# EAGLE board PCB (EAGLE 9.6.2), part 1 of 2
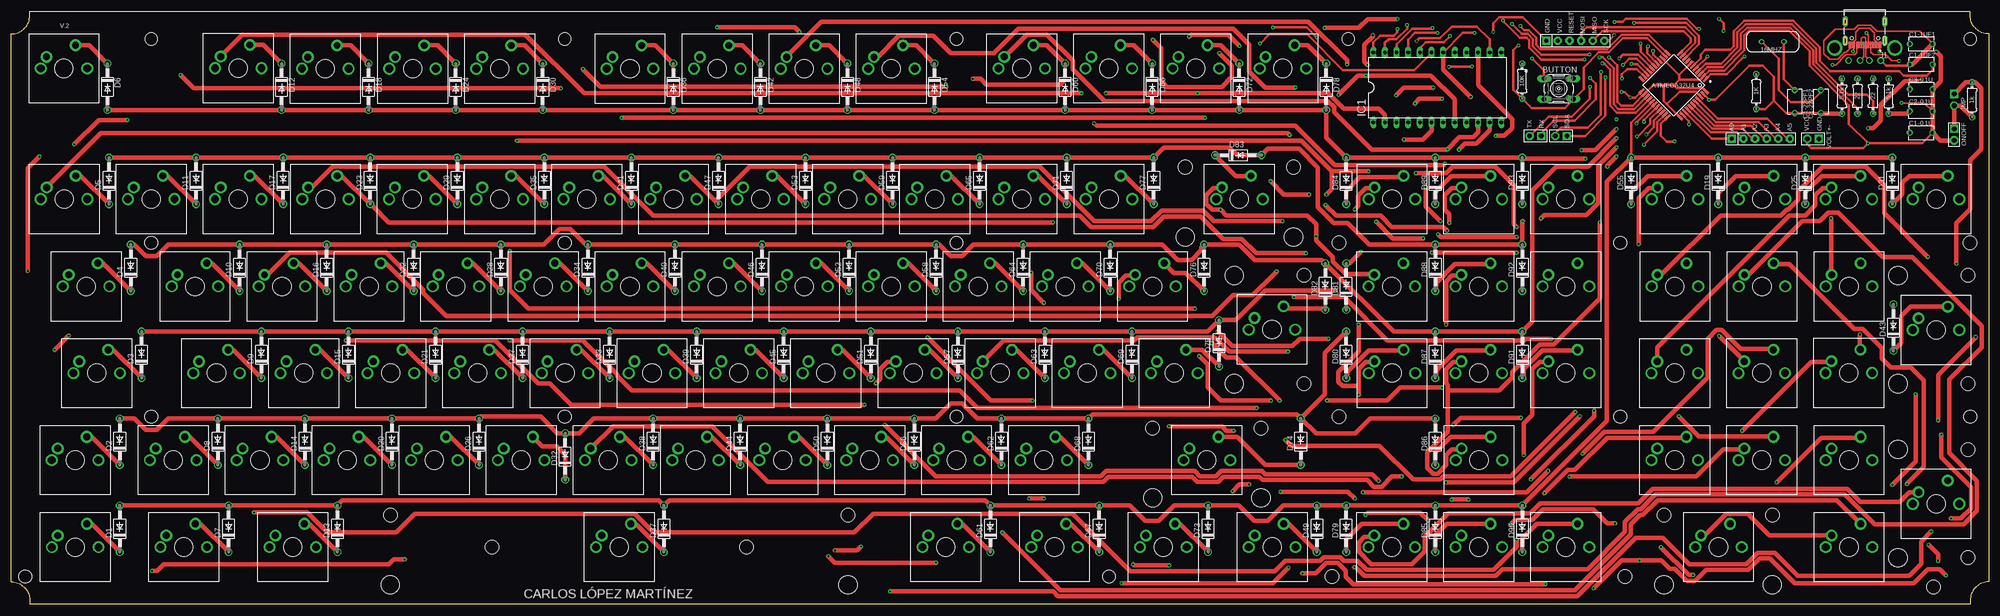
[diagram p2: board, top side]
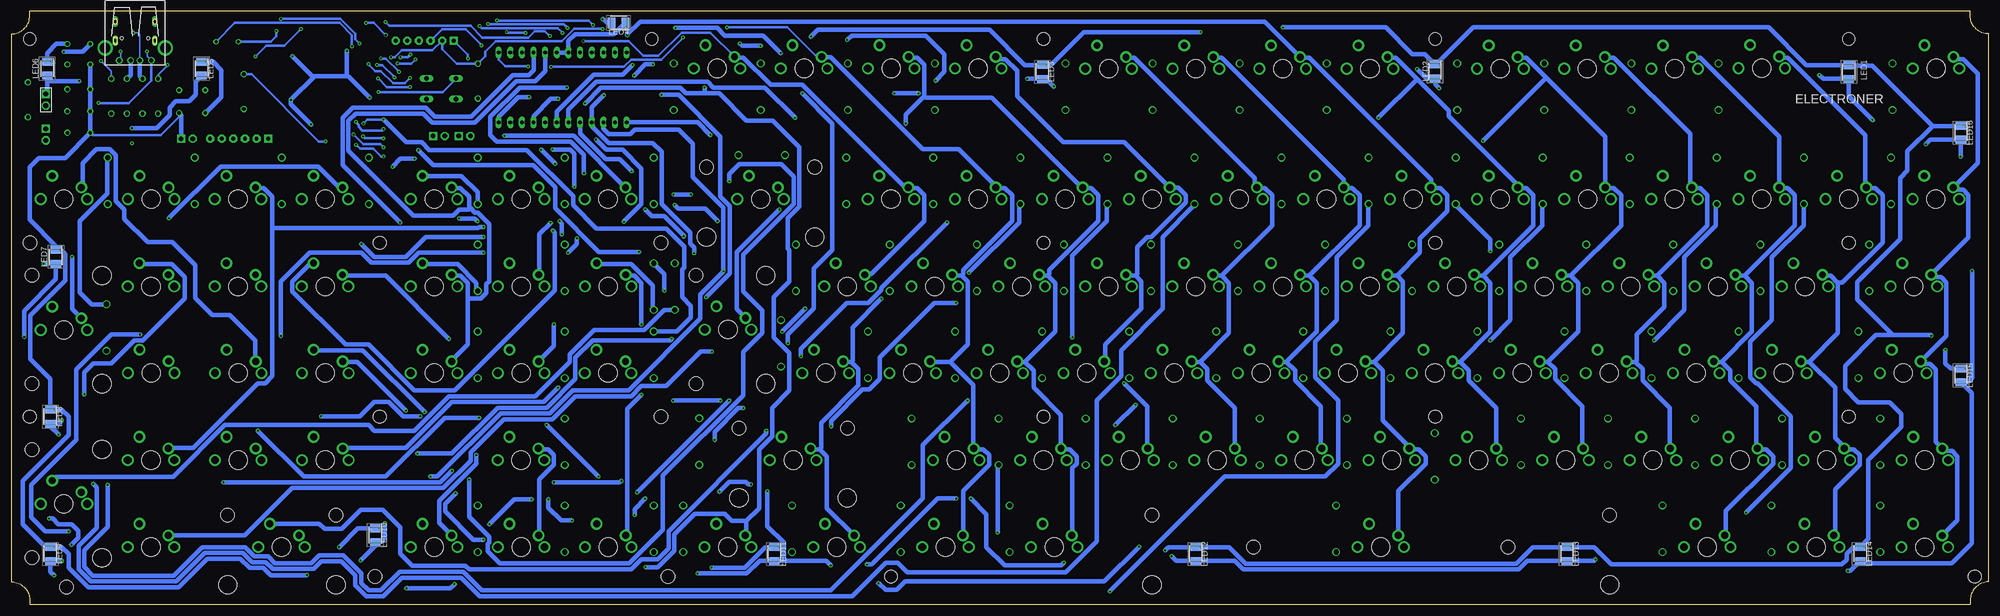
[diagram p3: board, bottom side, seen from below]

Size 431.5 x 129.5 mm. Coordinates in mm from the lower left corner, seen from the top.
Outline: 431.5,124.6 431.5,4.9 arc90 427.5,0.9 427.5,0 4,0 4,0.9 arc90 0,4.9 0,124.6 arc90 4,128.6 4,129.5 427.5,129.5 427.5,128.6 arc90 431.5,124.6
Copper layers (1*16): Top 0.035mm / dielectric 1.5mm / Bottom 0.035mm
Design rules "default *": minimum track width 0.3mm, minimum drill 0.35mm, track to track 3mil, track to pad 3mil, pad to pad 7mil, via to via 10mil, smd to smd 3mil, copper to edge 14mil, drill to drill 4mil, minimum pad ring 10mil, minimum via ring 8mil, stop-mask expansion 4mil, vias tented up to drill 0mil, thermal gap 10mil
Net classes: 0 default: width 0.203 mm
Holes 2.75 mm at 30.5,123.47 120.75,123.47 206.25,123.46 291.75,123.46 427.5,123.47
Holes 2.8 mm at 351.13,79 427.5,41 351.13,41 239.5,6.04 3,6.03 30.51,78.99 120.75,79 206.25,78.99 206.26,41 120.76,41 30.5,40.99
Holes 3 mm at 82.7,19.5 182.55,19.5 384.32,19.5 360.68,19.5 427,33.82 427,10.18 427,48.18 427,71.83 272.7,38.5 249.05,38.5 282.13,48.18 282.12,71.83 279.82,95.5 256.18,95.5 289.75,78.99 419.5,3.78 352.16,6.04 288.19,6.04 289.75,41 160.43,12.5 104.83,12.5 427.5,79
Holes 4 mm at 82.7,4.25 182.57,4.25 384.32,4.25 360.68,4.24 411.74,10.17 411.74,33.82 411.74,48.18 411.75,71.82 272.7,23.25 249.05,23.25 266.87,48.18 266.87,71.83 256.18,80.25 279.82,80.24

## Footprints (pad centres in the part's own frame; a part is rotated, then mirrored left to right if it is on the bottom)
SIP-100-06-32 = drill 0.813 pad 1.778 square: 1 -6.35,0 | drill 0.813 pad 1.778 octagon: 2 -3.81,0; 3 -1.27,0; 4 1.27,0; 5 3.81,0; 6 6.35,0
B3F-10XX = drill 1.016 long: 1 -3.251,2.261; 2 3.251,2.261; 3 -3.251,-2.261; 4 3.251,-2.261
CAP_RDE5C1H273J2M1H03A = drill 0.75 pad 1.15: 1 -2.5,0; 2 2.5,0
DO41-10 = drill 1.118: A 5.08,0; C -5.08,0
CHERRY-MX = drill 1.714 pad 1.93: P$3 -5.08,0; P$4 5.08,0 | drill 1.5 pad 2.54: SW1 -3.81,2.54; SW2 2.54,5.08 | hole 4: 0,0
DIL24-6 = drill 0.813 long: 1 -13.97,-7.62; 2 -11.43,-7.62; 3 -8.89,-7.62; 4 -6.35,-7.62; 5 -3.81,-7.62; 6 -1.27,-7.62; 7 1.27,-7.62; 8 3.81,-7.62; 9 6.35,-7.62; 10 8.89,-7.62; 11 11.43,-7.62; 12 13.97,-7.62; 13 13.97,7.62; 14 11.43,7.62; 15 8.89,7.62; 16 6.35,7.62; 17 3.81,7.62; 18 1.27,7.62; 19 -1.27,7.62; 20 -3.81,7.62; 21 -6.35,7.62; 22 -8.89,7.62; 23 -11.43,7.62; 24 -13.97,7.62
HRO_TYPE-C-31-M-12 = smd 0.6 x 1.45: A1B12 -3.25,5.095; A4B9 -2.45,5.095; B1A12 3.25,5.095; B4A9 2.45,5.095 | smd 0.3 x 1.45: A5 -1.25,5.095; A6 -0.25,5.095; A7 0.25,5.095; A8 1.25,5.095; B5 1.75,5.095; B6 0.75,5.095; B7 -0.75,5.095; B8 -1.75,5.095 | drill 0.65 pad 1.05 long: S1 -4.32,4.18; S2 4.32,4.18; S3 -4.32,0; S4 4.32,0 | hole 0.7: -2.89,3.65; 2.89,3.65
LEDM3528X200N = smd 1.65 x 2.25: 1 -1.5,0; 2 1.5,0
SIP-100-02-40 = drill 1.016 pad 1.778 square: 1 -1.27,0 | drill 1.016 pad 1.778 octagon: 2 1.27,0
0204/7 = drill 0.813 octagon: 1 -3.81,0; 2 3.81,0
QFP80P1200X1200X120-44N = smd 1.5 x 0.5: 1 -5.9,4; 2 -5.9,3.2; 3 -5.9,2.4; 4 -5.9,1.6; 5 -5.9,0.8; 6 -5.9,0; 7 -5.9,-0.8; 8 -5.9,-1.6; 9 -5.9,-2.4; 10 -5.9,-3.2; 11 -5.9,-4; 23 5.9,-4; 24 5.9,-3.2; 25 5.9,-2.4; 26 5.9,-1.6; 27 5.9,-0.8; 28 5.9,0; 29 5.9,0.8; 30 5.9,1.6; 31 5.9,2.4; 32 5.9,3.2; 33 5.9,4 | smd 0.5 x 1.5: 12 -4,-5.9; 13 -3.2,-5.9; 14 -2.4,-5.9; 15 -1.6,-5.9; 16 -0.8,-5.9; 17 0,-5.9; 18 0.8,-5.9; 19 1.6,-5.9; 20 2.4,-5.9; 21 3.2,-5.9; 22 4,-5.9; 34 4,5.9; 35 3.2,5.9; 36 2.4,5.9; 37 1.6,5.9; 38 0.8,5.9; 39 0,5.9; 40 -0.8,5.9; 41 -1.6,5.9; 42 -2.4,5.9; 43 -3.2,5.9; 44 -4,5.9
USB-A-H = drill 0.914: D+ 2.718,-1.003; D- 2.718,1.003; GND 2.718,-3.493; VBUS 2.718,3.493 | drill 2.311: P$5 0,-6.566; P$6 0,6.566
XTAL_ECS-160-20-4X = drill 0.63 pad 1.03: 1 -2.44,0; 2 2.44,0

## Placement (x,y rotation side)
ANALOG  Boot  [SIP-100-06-32]  381.8,101.7 0 top
BUTTON  [B3F-10XX]  337.7,112.6 0 top
C1-0.1U  RDE5C1H273J2M1H03A  [CAP_RDE5C1H273J2M1H03A]  416.8,103 180 top
C1-1UF1  RDE5C1H273J2M1H03A  [CAP_RDE5C1H273J2M1H03A]  416.8,122.4 0 top
C1-1UF2  RDE5C1H273J2M1H03A  [CAP_RDE5C1H273J2M1H03A]  416.8,117.9 180 top
C1-22PF1  RDE5C1H273J2M1H03A  [CAP_RDE5C1H273J2M1H03A]  389.2,109.8 270 top
C1-22PF2  RDE5C1H273J2M1H03A  [CAP_RDE5C1H273J2M1H03A]  394.9,109.8 270 top
C2-0.1U  RDE5C1H273J2M1H03A  [CAP_RDE5C1H273J2M1H03A]  416.8,107.7 180 top
C3-0.1U  RDE5C1H273J2M1H03A  [CAP_RDE5C1H273J2M1H03A]  416.8,112.5 180 top
D1  1N4004  [DO41-10]  23.65,16.5 90 top
D2  1N4004  [DO41-10]  23.65,35.5 90 top
D3  1N4004  [DO41-10]  28.4,54.5 90 top
D4  1N4004  [DO41-10]  26.05,73.5 90 top
D5  1N4004  [DO41-10]  21.3,92.5 90 top
D6  1N4004  [DO41-10]  20.95,113.05 270 top
D7  1N4004  [DO41-10]  47.4,16.5 90 top
D8  1N4004  [DO41-10]  45.05,35.5 90 top
D9  1N4004  [DO41-10]  54.55,54.5 90 top
D10  1N4004  [DO41-10]  49.8,73.5 90 top
D11  1N4004  [DO41-10]  40.3,92.5 90 top
D12  1N4004  [DO41-10]  58.95,113.05 270 top
D13  1N4004  [DO41-10]  71.15,16.5 90 top
D14  1N4004  [DO41-10]  64.05,35.5 90 top
D15  1N4004  [DO41-10]  73.55,54.5 90 top
D16  1N4004  [DO41-10]  68.8,73.5 90 top
D17  1N4004  [DO41-10]  59.3,92.5 90 top
D18  1N4004  [DO41-10]  77.95,113.05 270 top
D19  1N4004  [DO41-10]  372.5,92.5 90 top
D20  1N4004  [DO41-10]  83.05,35.5 90 top
D21  1N4004  [DO41-10]  92.55,54.5 90 top
D22  1N4004  [DO41-10]  87.8,73.5 90 top
D23  1N4004  [DO41-10]  78.3,92.5 90 top
D24  1N4004  [DO41-10]  96.95,113.05 270 top
D25  1N4004  [DO41-10]  391.5,92.5 90 top
D26  1N4004  [DO41-10]  102.05,35.5 90 top
D27  1N4004  [DO41-10]  111.55,54.5 90 top
D28  1N4004  [DO41-10]  106.8,73.5 90 top
D29  1N4004  [DO41-10]  97.3,92.5 90 top
D30  1N4004  [DO41-10]  115.95,113.05 270 top
D31  1N4004  [DO41-10]  410.5,92.5 90 top
D32  1N4004  [DO41-10]  120.85,32.3 90 top
D33  1N4004  [DO41-10]  130.55,54.5 90 top
D34  1N4004  [DO41-10]  125.8,73.5 90 top
D35  1N4004  [DO41-10]  116.3,92.5 90 top
D36  1N4004  [DO41-10]  144.45,113.05 270 top
D37  1N4004  [DO41-10]  142.4,16.5 90 top
D38  1N4004  [DO41-10]  140.05,35.5 90 top
D39  1N4004  [DO41-10]  149.55,54.5 90 top
D40  1N4004  [DO41-10]  144.8,73.5 90 top
D41  1N4004  [DO41-10]  135.3,92.5 90 top
D42  1N4004  [DO41-10]  163.45,113.05 270 top
D43  1N4004  [DO41-10]  410.75,60.45 90 top
D44  1N4004  [DO41-10]  159.05,35.5 90 top
D45  1N4004  [DO41-10]  168.55,54.5 90 top
D46  1N4004  [DO41-10]  163.8,73.5 90 top
D47  1N4004  [DO41-10]  154.3,92.5 90 top
D48  1N4004  [DO41-10]  182.45,113.05 270 top
D49  1N4004  [DO41-10]  284.9,16.5 90 top
D50  1N4004  [DO41-10]  178.05,35.5 90 top
D51  1N4004  [DO41-10]  187.55,54.5 90 top
D52  1N4004  [DO41-10]  182.8,73.5 90 top
D53  1N4004  [DO41-10]  173.3,92.5 90 top
D54  1N4004  [DO41-10]  201.45,113.05 270 top
D55  1N4004  [DO41-10]  353.5,92.5 90 top
D56  1N4004  [DO41-10]  197.05,35.5 90 top
D57  1N4004  [DO41-10]  206.55,54.5 90 top
D58  1N4004  [DO41-10]  201.8,73.5 90 top
D59  1N4004  [DO41-10]  192.3,92.5 90 top
D60  1N4004  [DO41-10]  229.95,113.05 270 top
D61  1N4004  [DO41-10]  213.65,16.5 90 top
D62  1N4004  [DO41-10]  216.05,35.5 90 top
D63  1N4004  [DO41-10]  225.55,54.5 90 top
D64  1N4004  [DO41-10]  220.8,73.5 90 top
D65  1N4004  [DO41-10]  211.3,92.5 90 top
D66  1N4004  [DO41-10]  248.95,113.05 270 top
D67  1N4004  [DO41-10]  237.4,16.5 90 top
D68  1N4004  [DO41-10]  235.05,35.5 90 top
D69  1N4004  [DO41-10]  244.55,54.5 90 top
D70  1N4004  [DO41-10]  239.8,73.5 90 top
D71  1N4004  [DO41-10]  230.3,92.5 90 top
D72  1N4004  [DO41-10]  267.95,113.05 270 top
D73  1N4004  [DO41-10]  261.15,16.5 90 top
D74  1N4004  [DO41-10]  281.4,35.55 90 top
D75  1N4004  [DO41-10]  263.55,57 90 top
D76  1N4004  [DO41-10]  260.3,73.5 90 top
D77  1N4004  [DO41-10]  249.3,92.5 90 top
D78  1N4004  [DO41-10]  286.95,113.05 270 top
D79  1N4004  [DO41-10]  291.3,16.5 90 top
D80  1N4004  [DO41-10]  291.3,54.5 90 top
D81  1N4004  [DO41-10]  291.3,69.4 90 top
D82  1N4004  [DO41-10]  286.75,69.4 90 top
D83  1N4004  [DO41-10]  267.75,98.1 0 top
D84  1N4004  [DO41-10]  291.3,92.5 90 top
D85  1N4004  [DO41-10]  310.75,16.5 90 top
D86  1N4004  [DO41-10]  310.75,35.5 90 top
D87  1N4004  [DO41-10]  310.75,54.5 90 top
D88  1N4004  [DO41-10]  310.75,73.5 90 top
D89  1N4004  [DO41-10]  310.75,92.5 90 top
D90  1N4004  [DO41-10]  329.75,16.5 90 top
D91  1N4004  [DO41-10]  329.75,54.5 90 top
D92  1N4004  [DO41-10]  329.75,73.5 90 top
D93  1N4004  [DO41-10]  329.75,92.5 90 top
DUPLICADO1  CHERRY-MX  [CHERRY-MX]  363,31.5 0 top
DUPLICADO2  CHERRY-MX  [CHERRY-MX]  382,31.5 0 top
DUPLICADO3  CHERRY-MX  [CHERRY-MX]  401.05,31.5 0 top
DUPLICADO4  CHERRY-MX  [CHERRY-MX]  363,50.5 0 top
DUPLICADO5  CHERRY-MX  [CHERRY-MX]  382,50.5 0 top
DUPLICADO6  CHERRY-MX  [CHERRY-MX]  401,50.55 0 top
DUPLICADO7  CHERRY-MX  [CHERRY-MX]  363.05,69.45 0 top
DUPLICADO8  CHERRY-MX  [CHERRY-MX]  382.05,69.45 0 top
DUPLICADO9  CHERRY-MX  [CHERRY-MX]  401.05,69.45 0 top
DUPLICADO10  CHERRY-MX  [CHERRY-MX]  372.55,12.5 0 top
ENTERDUPLICADO  CHERRY-MX  [CHERRY-MX]  420.05,21.95 0 top
IC1  74154N  [DIL24-6]  311.2,112.9 0 top
J1  TYPE-C-31-M-12  [HRO_TYPE-C-31-M-12]  404.5,127.3 180 top
J3  Boot  [SIP-100-06-32]  341.3,123.1 0 top
LED1  ASMM-CA03-AS402  [LEDM3528X200N]  30.49,116.26 270 bottom
LED2  ASMM-CA03-AS402  [LEDM3528X200N]  120.8,116.4 270 bottom
LED3  ASMM-CA03-AS402  [LEDM3528X200N]  206.5,116.3 270 bottom
LED4  ASMM-CA03-AS402  [LEDM3528X200N]  299,127 180 bottom
LED5  ASMM-CA03-AS402  [LEDM3528X200N]  390,117 270 bottom
LED6  ASMM-CA03-AS402  [LEDM3528X200N]  423.7,117 270 bottom
LED7  ASMM-CA03-AS402  [LEDM3528X200N]  421.8,75.9 270 bottom
LED8  ASMM-CA03-AS402  [LEDM3528X200N]  423,41 270 bottom
LED9  ASMM-CA03-AS402  [LEDM3528X200N]  423,11 270 bottom
LED10  ASMM-CA03-AS402  [LEDM3528X200N]  352.1,15.1 270 bottom
LED11  ASMM-CA03-AS402  [LEDM3528X200N]  265,11 270 bottom
LED12  ASMM-CA03-AS402  [LEDM3528X200N]  173,11 270 bottom
LED13  ASMM-CA03-AS402  [LEDM3528X200N]  92,11 270 bottom
LED14  ASMM-CA03-AS402  [LEDM3528X200N]  28,11 270 bottom
LED15  ASMM-CA03-AS402  [LEDM3528X200N]  6,50 270 bottom
LED16  ASMM-CA03-AS402  [LEDM3528X200N]  6,103 270 bottom
LEDSJUMPER  F-1X02-SIP-100-40  [SIP-100-02-40]  424,110.2 270 bottom
ONOFF  F-1X02-SIP-100-40  [SIP-100-02-40]  424,102.6 270 top
PUNTODUPLICADO  CHERRY-MX  [CHERRY-MX]  401.05,12.5 0 top
R1  22  [0204/7]  406.3,111 90 top
R2  22  [0204/7]  402.9,111 90 top
R3  1K  [0204/7]  427.9,110.2 270 top
R4  1K  [0204/7]  380.8,112 90 top
R5  10K  [0204/7]  329.7,114.3 270 top
R6  5.1K  [0204/7]  409.7,111 270 top
R7  5.1K  [0204/7]  399.5,111 270 top
RXTX  F-1X02-SIP-100-40  [SIP-100-02-40]  332.6,102.3 180 top
SD  F-1X02-SIP-100-40  [SIP-100-02-40]  338.2,102.3 180 top
U1  ATMEGA32U4-AU  [QFP80P1200X1200X120-44N]  362.8,113.4 225 top
U$1  CHERRY-MX  [CHERRY-MX]  13.91,12.49 0 top
U$2  CHERRY-MX  [CHERRY-MX]  13.9,31.5 0 top
U$3  CHERRY-MX  [CHERRY-MX]  18.6,50.5 0 top
U$4  CHERRY-MX  [CHERRY-MX]  16.3,69.45 0 top
U$5  CHERRY-MX  [CHERRY-MX]  11.5,88.5 0 top
U$6  CHERRY-MX  [CHERRY-MX]  11.45,117.05 0 top
U$7  CHERRY-MX  [CHERRY-MX]  37.6,12.5 0 top
U$8  CHERRY-MX  [CHERRY-MX]  35.3,31.5 0 top
U$9  CHERRY-MX  [CHERRY-MX]  44.75,50.5 0 top
U$10  CHERRY-MX  [CHERRY-MX]  40.05,69.45 0 top
U$11  CHERRY-MX  [CHERRY-MX]  30.5,88.5 0 top
U$12  CHERRY-MX  [CHERRY-MX]  49.5,117.1 0 top
U$13  CHERRY-MX  [CHERRY-MX]  61.4,12.5 0 top
U$14  CHERRY-MX  [CHERRY-MX]  54.25,31.5 0 top
U$15  CHERRY-MX  [CHERRY-MX]  63.8,50.5 0 top
U$16  CHERRY-MX  [CHERRY-MX]  59.05,69.45 0 top
U$17  CHERRY-MX  [CHERRY-MX]  49.5,88.5 0 top
U$18  CHERRY-MX  [CHERRY-MX]  68.5,117 0 top
U$19  CHERRY-MX  [CHERRY-MX]  382.05,88.5 0 top
U$20  CHERRY-MX  [CHERRY-MX]  73.25,31.5 0 top
U$21  CHERRY-MX  [CHERRY-MX]  82.8,50.5 0 top
U$22  CHERRY-MX  [CHERRY-MX]  78.05,69.45 0 top
U$23  CHERRY-MX  [CHERRY-MX]  68.55,88.5 0 top
U$24  CHERRY-MX  [CHERRY-MX]  87.55,117 0 top
U$25  CHERRY-MX  [CHERRY-MX]  401,88.5 0 top
U$26  CHERRY-MX  [CHERRY-MX]  92.3,31.5 0 top
U$27  CHERRY-MX  [CHERRY-MX]  101.75,50.5 0 top
U$28  CHERRY-MX  [CHERRY-MX]  97,69.45 0 top
U$29  CHERRY-MX  [CHERRY-MX]  87.5,88.5 0 top
U$30  CHERRY-MX  [CHERRY-MX]  106.55,117 0 top
U$31  CHERRY-MX  [CHERRY-MX]  420.05,88.5 0 top
U$32  CHERRY-MX  [CHERRY-MX]  111.25,31.5 0 top
U$33  CHERRY-MX  [CHERRY-MX]  120.8,50.5 0 top
U$34  CHERRY-MX  [CHERRY-MX]  116.05,69.45 0 top
U$35  CHERRY-MX  [CHERRY-MX]  106.55,88.5 0 top
U$36  CHERRY-MX  [CHERRY-MX]  135,117 0 top
U$37  CHERRY-MX  [CHERRY-MX]  132.65,12.5 0 top
U$38  CHERRY-MX  [CHERRY-MX]  130.25,31.5 0 top
U$39  CHERRY-MX  [CHERRY-MX]  139.8,50.5 0 top
U$40  CHERRY-MX  [CHERRY-MX]  135,69.45 0 top
U$41  CHERRY-MX  [CHERRY-MX]  125.55,88.5 0 top
U$42  CHERRY-MX  [CHERRY-MX]  154.05,117 0 top
U$43  CHERRY-MX  [CHERRY-MX]  420.05,59.95 0 top
U$44  CHERRY-MX  [CHERRY-MX]  149.3,31.5 0 top
U$45  CHERRY-MX  [CHERRY-MX]  158.75,50.5 0 top
U$46  CHERRY-MX  [CHERRY-MX]  154.05,69.45 0 top
U$47  CHERRY-MX  [CHERRY-MX]  144.5,88.5 0 top
U$48  CHERRY-MX  [CHERRY-MX]  173,117 0 top
U$49  CHERRY-MX  [CHERRY-MX]  275.15,12.5 0 top
U$50  CHERRY-MX  [CHERRY-MX]  168.3,31.5 0 top
U$51  CHERRY-MX  [CHERRY-MX]  177.75,50.5 0 top
U$52  CHERRY-MX  [CHERRY-MX]  173.05,69.45 0 top
U$53  CHERRY-MX  [CHERRY-MX]  163.5,88.5 0 top
U$54  CHERRY-MX  [CHERRY-MX]  192.05,117 0 top
U$55  CHERRY-MX  [CHERRY-MX]  363.05,88.5 0 top
U$56  CHERRY-MX  [CHERRY-MX]  187.3,31.5 0 top
U$57  CHERRY-MX  [CHERRY-MX]  196.8,50.5 0 top
U$58  CHERRY-MX  [CHERRY-MX]  192.05,69.45 0 top
U$59  CHERRY-MX  [CHERRY-MX]  182.5,88.5 0 top
U$60  CHERRY-MX  [CHERRY-MX]  220.5,117.05 0 top
U$61  CHERRY-MX  [CHERRY-MX]  203.9,12.5 0 top
U$62  CHERRY-MX  [CHERRY-MX]  206.25,31.5 0 top
U$63  CHERRY-MX  [CHERRY-MX]  215.8,50.5 0 top
U$64  CHERRY-MX  [CHERRY-MX]  211,69.45 0 top
U$65  CHERRY-MX  [CHERRY-MX]  201.5,88.5 0 top
U$66  CHERRY-MX  [CHERRY-MX]  239.5,117.05 0 top
U$67  CHERRY-MX  [CHERRY-MX]  227.65,12.5 0 top
U$68  CHERRY-MX  [CHERRY-MX]  225.3,31.5 0 top
U$69  CHERRY-MX  [CHERRY-MX]  234.8,50.5 0 top
U$70  CHERRY-MX  [CHERRY-MX]  230,69.45 0 top
U$71  CHERRY-MX  [CHERRY-MX]  220.5,88.5 0 top
U$72  CHERRY-MX  [CHERRY-MX]  258.5,117.05 0 top
U$73  CHERRY-MX  [CHERRY-MX]  251.4,12.5 0 top
U$74  CHERRY-MX  [CHERRY-MX]  260.9,31.5 0 top
U$75  CHERRY-MX  [CHERRY-MX]  253.8,50.5 0 top
U$76  CHERRY-MX  [CHERRY-MX]  249.05,69.45 0 top
U$77  CHERRY-MX  [CHERRY-MX]  239.55,88.5 0 top
U$78  CHERRY-MX  [CHERRY-MX]  277.5,117.05 0 top
U$79  CHERRY-MX  [CHERRY-MX]  301.25,12.5 0 top
U$80  CHERRY-MX  [CHERRY-MX]  301.3,50.5 0 top
U$81  CHERRY-MX  [CHERRY-MX]  301.25,69.45 0 top
U$82  CHERRY-MX  [CHERRY-MX]  275.1,60 0 top
U$83  CHERRY-MX  [CHERRY-MX]  268,88.5 0 top
U$84  CHERRY-MX  [CHERRY-MX]  301.3,88.5 0 top
U$85  CHERRY-MX  [CHERRY-MX]  320.25,12.5 0 top
U$86  CHERRY-MX  [CHERRY-MX]  320.3,31.5 0 top
U$87  CHERRY-MX  [CHERRY-MX]  320.25,50.5 0 top
U$88  CHERRY-MX  [CHERRY-MX]  320.25,69.45 0 top
U$89  CHERRY-MX  [CHERRY-MX]  320.25,88.5 0 top
U$90  CHERRY-MX  [CHERRY-MX]  339.25,12.5 0 top
U$91  CHERRY-MX  [CHERRY-MX]  339.25,50.5 0 top
U$92  CHERRY-MX  [CHERRY-MX]  339.25,69.45 0 top
U$93  CHERRY-MX  [CHERRY-MX]  339.25,88.5 0 top
VOLT+-  F-1X02-SIP-100-40  [SIP-100-02-40]  393.2,101.7 180 top
X2  USB-A-H  [USB-A-H]  404.48,121.5 270 bottom
Y1  ECS-160-20-4X  [XTAL_ECS-160-20-4X]  384.4,122.9 180 top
